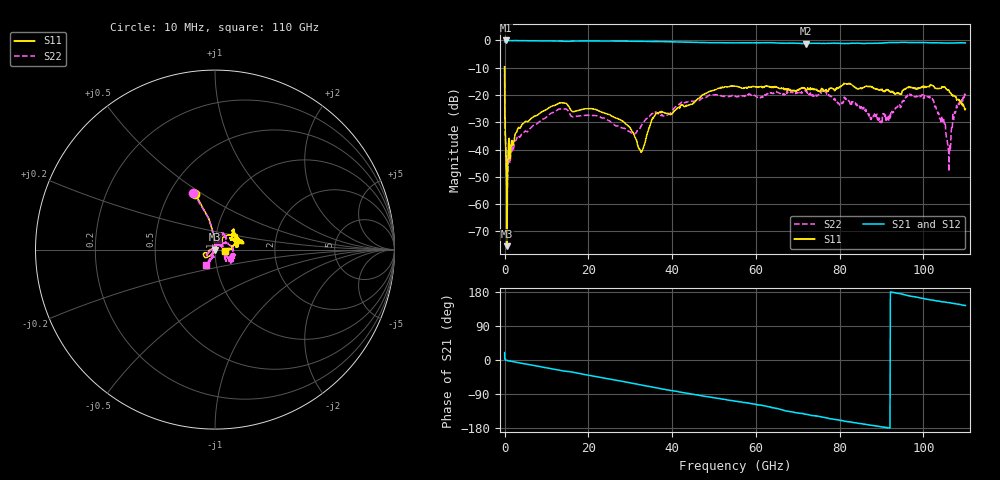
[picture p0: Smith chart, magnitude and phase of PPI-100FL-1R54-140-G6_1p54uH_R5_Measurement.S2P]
! Data measured by Modelithics Inc.  support@modelithics.com  813-866-6335  Tampa FL USA June 2025
! PPI-100FL-1R54-140-G6_1p54uH measured on 5-mil thick RO3003G2 board, mounted in 2-port shunt configuration on a 50-ohm transmission line
# GHz S RI R 50.0
!freq ReS11 ImS11 ReS21 ImS21 ReS12 ImS12 ReS22 ImS22
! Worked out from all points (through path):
!   1207 points, 10 MHz to 110 GHz, reference 50 ohm
!   highest |S21| = -0.01 dB at 300 MHz (marker M1); lowest = -1.2 dB at 71.9 GHz (marker M2)
!   group delay of S21, straight-line fit = 5.46 ps
!   lowest |S11| = -75.4 dB at 591.3 MHz (marker M3), VSWR 1.00, Z = 50 - j0.00208 ohm
!   |S11| at or under -10 dB: 10.65 MHz to end of sweep
!   |S22| runs from -61.5 to -9.4 dB; largest |S21 - S12| = 0.077
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0.01  -0.1102 0.3106  0.8848 0.3138  0.8847 0.3137  -0.1205 0.3159
0.2  -0.000989 0.0168  0.9986 0.00974  0.9984 0.00973  -0.00136 0.0168
0.3  -0.00051 0.00967  0.9987 -0.000738  0.9986 -0.000762  -0.000964 0.00973
0.5912664  0.000168 -2.08e-05  0.9982 -0.0199  0.9981 -0.0198  -0.000828 0.000165
0.9796215  -0.00525 -0.013  0.9906 -0.0437  0.9905 -0.0435  -0.00826 -0.0103
1.465066  -0.00356 -0.00861  0.9925 -0.0542  0.9924 -0.0539  -0.00468 -0.00655
4.766084  -0.0177 -0.026  0.9702 -0.172  0.9703 -0.1709  -0.0123 -0.0173
13.11572  -0.0567 -0.0432  0.8646 -0.4436  0.8649 -0.4432  -0.0379 -0.0402
18.35852  -0.0441 -0.0313  0.7847 -0.5837  0.7846 -0.5838  -0.0331 -0.0258
28.16448  -0.0327 -0.00475  0.5375 -0.8116  0.5362 -0.8124  -0.0248 -0.000271
32.53348  -0.00405 0.008  0.3988 -0.8815  0.3944 -0.8834  0.00311 0.0264
36.7083  0.0191 0.0435  0.2567 -0.9204  0.2532 -0.9213  0.0428 0.0136
55.05808  0.1223 0.0776  -0.2905 -0.8567  -0.2839 -0.8589  0.0872 -0.0368
71.9  0.1219 0.0307  -0.6971 -0.5249  -0.6888 -0.5515  0.1058 -0.0484
73.4  0.1231 0.0404  -0.7417 -0.4865  -0.7051 -0.53  0.083 -0.0506
91.7  0.1101 0.049  -0.9098 -0.0172  -0.913 -0.0144  0.0105 0.033
96.4  0.1031 0.089  -0.9017 0.1662  -0.9076 0.1321  0.0396 0.0899
101.5  0.0946 0.1062  -0.8455 0.3243  -0.8553 0.3006  0.0637 0.0619
104.7  0.1289 0.0574  -0.8025 0.3992  -0.8054 0.4001  0.0126 0.035
106  0.1173 0.0374  -0.786 0.428  -0.786 0.4309  0.00451 0.00768
107.6  0.0931 0.00669  -0.7674 0.465  -0.7687 0.469  -0.0194 -0.0426
110  0.0538 -0.0101  -0.7258 0.5343  -0.731 0.5317  -0.0499 -0.0849
